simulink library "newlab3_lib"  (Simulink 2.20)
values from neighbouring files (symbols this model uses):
  h = 0.05    [initlab3.m]
undefined symbols (not defined in the file or in its folder): A, AIno, AOno, B, C, D, R, S, T, Ts, Xo

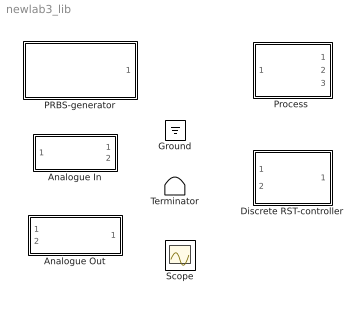
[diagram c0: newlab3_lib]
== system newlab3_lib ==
  Analogue In : Subsystem  mask(AnalogueIOBlock){h=h, AIno=AIno}
      mask prompts: h "Sample period"; AIno "Input port number"
      mask help: Analogue input block for use on PC running Linux.
  Analogue Out : Subsystem  mask(AnalogueIOBlock){h=h, AOno=AOno}
      mask prompts: h "Sample period"; AOno "Output port number"
      mask help: Analogue output block for use on PC running Linux
  Discrete RST-controller : Subsystem  mask(ControllerMaskBlock){R=R, S=S, T=T, h=h}
      mask prompts: R "R-polynomial"; S "S-polynomial"; T "T-polynomial"; h "Sample period"
      mask help: Discrete RST-controller (forward shift) R(q)u = -S(q)y + T(q)y_ref
  Ground : Ground
  PRBS-generator : Subsystem  mask(PRBSblockMask){h=h, N=5, Amp=2, offset=0, seed=0}
      mask prompts: h "Sample time (h)"; N "PRBS period (N)"; Amp "Amplitude"; seed "Random seed"
      mask help: A (P)RBS-generator
  "Process " : Subsystem  mask(SIMO Process){AOu=0, AIy=0, AIu=1, h=h}
      mask prompts: AOu "AO  u"; AIy "AI y"; AIu "AI u"; h "Sample Period"
      mask help: Process communication block. For use with Linux on PC with I/O.
  Scope : Scope
  Terminator : Terminator

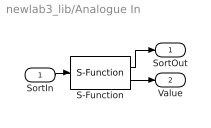
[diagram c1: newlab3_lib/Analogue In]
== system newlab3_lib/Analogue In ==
  SortIn : Inport  Port=1  PortWidth=-1  SampleTime=-1
  S-Function : S-Function  FunctionName=analogin  Parameters=h AIno  PortCounts=[]  SFunctionModules=''
  SortOut : Outport  Port=1  InitialOutput=0
  Value : Outport  Port=2  InitialOutput=0
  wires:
  S-Function/2 -> Value/1
  SortIn/1 -> S-Function/1
  S-Function/1 -> SortOut/1

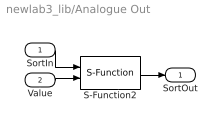
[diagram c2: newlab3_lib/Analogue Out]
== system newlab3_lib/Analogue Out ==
  SortIn : Inport  Port=1  PortWidth=-1  SampleTime=-1
  Value : Inport  Port=2  PortWidth=-1  SampleTime=-1
  S-Function2 : S-Function  FunctionName=analogout  Parameters=h AOno  PortCounts=[]  SFunctionModules=''
  SortOut : Outport  Port=1  InitialOutput=0
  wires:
  Value/1 -> S-Function2/2
  S-Function2/1 -> SortOut/1
  SortIn/1 -> S-Function2/1

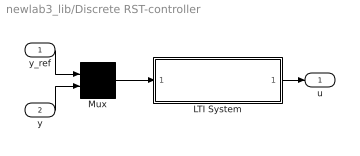
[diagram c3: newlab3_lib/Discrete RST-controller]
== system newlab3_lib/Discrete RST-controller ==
  y_ref : Inport  Port=1  PortWidth=-1  SampleTime=-1
  y : Inport  Port=2  PortWidth=-1  SampleTime=-1
  LTI System : Subsystem  mask(LTI Block){sys=ss(tf({T, -S},{R,R},h)), IC=0}
      mask prompts: sys "LTI system variable"; IC "Initial states   (state space only)"
      mask help: The LTI System Block accepts both continuous and discrete LTI objects as defined in the Control System Toolbox. Transfer function, state space, and zero/pole/gain formats are all supported in this block. Note: For multi-input systems, the input delays must be either all positive or all zero. Note: Initial states are only meaningful for state-space systems.
      mask init:
      | sysname='xxx';
      | [A,B,C,D,Xo,Td,Ts,sysname]=ltimask( 'InitializeVars',gcb,sys,IC,&1,&2);
      | ltimask( 'UpdateDiagram',gcb,sys,Td);
  Mux : Mux  Inputs=2
  u : Outport  Port=1  InitialOutput=0
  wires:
  y/1 -> Mux/2
  LTI System/1(Out1) -> u/1
  y_ref/1 -> Mux/1
  Mux/1 -> LTI System/1(In1)

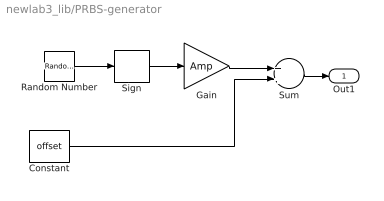
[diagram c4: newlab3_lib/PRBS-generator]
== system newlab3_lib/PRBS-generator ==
  Constant : Constant  Value=offset
  Gain : Gain  Gain=Amp
  Random Number : RandomNumber  Mean=0  Variance=1  Seed=seed  SampleTime=h*N
  Sign : Signum
  Sum : Sum  Inputs=++
  Out1 : Outport  Port=1  InitialOutput=0
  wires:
  Random Number/1 -> Sign/1
  Sign/1 -> Gain/1
  Gain/1 -> Sum/1
  Constant/1 -> Sum/2
  Sum/1 -> Out1/1

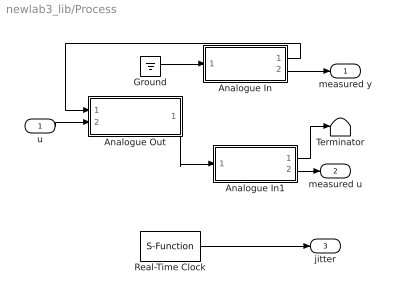
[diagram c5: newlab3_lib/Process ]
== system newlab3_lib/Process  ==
  u : Inport  Port=1  PortWidth=-1  SampleTime=-1
  Analogue In : Subsystem  mask(AnalogueIOBlock){h=h, AIy=AIy}
      mask prompts: h "Sample period"; AIy "Input port number"
      mask help: Analogue input block for use on PC running Linux.
  Analogue In1 : Subsystem  mask(AnalogueIOBlock){h=h, AIu=AIu}
      mask prompts: h "Sample period"; AIu "Input port number"
      mask help: Analogue input block for use on PC running Linux.
  Analogue Out : Subsystem  mask(AnalogueIOBlock){h=h, AOu=AOu}
      mask prompts: h "Sample period"; AOu "Output port number"
      mask help: Analogue output block for use on PC running Linux
  Ground : Ground
  Real-Time Clock : S-Function  FunctionName=timer  Parameters=h  PortCounts=[]  SFunctionModules=''
  Terminator : Terminator
  measured y : Outport  Port=1
  measured u : Outport  Port=2
  jitter : Outport  Port=3
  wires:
  Analogue In/1(SortOut) -> Analogue Out/1(SortIn)
  u/1 -> Analogue Out/2(Value)
  Real-Time Clock/1 -> jitter/1
  Analogue In/2(Value) -> measured y/1
  Ground/1 -> Analogue In/1(SortIn)
  Analogue In1/1(SortOut) -> Terminator/1
  Analogue In1/2(Value) -> measured u/1
  Analogue Out/1(SortOut) -> Analogue In1/1(SortIn)

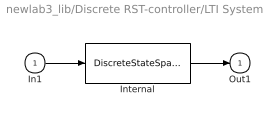
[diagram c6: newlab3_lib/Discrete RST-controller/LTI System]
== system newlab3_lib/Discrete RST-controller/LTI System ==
  In1 : Inport  Port=1  PortWidth=-1  SampleTime=-1
  Internal : DiscreteStateSpace  A=A  B=B  C=C  D=D  X0=Xo  SampleTime=Ts
  Out1 : Outport  Port=1  InitialOutput=0
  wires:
  In1/1 -> Internal/1
  Internal/1 -> Out1/1

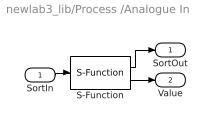
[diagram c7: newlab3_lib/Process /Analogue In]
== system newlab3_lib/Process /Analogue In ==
  SortIn : Inport  Port=1  PortWidth=-1  SampleTime=-1
  S-Function : S-Function  FunctionName=analogin  Parameters=h AIy  PortCounts=[]  SFunctionModules=''
  SortOut : Outport  Port=1  InitialOutput=0
  Value : Outport  Port=2  InitialOutput=0
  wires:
  S-Function/1 -> SortOut/1
  SortIn/1 -> S-Function/1
  S-Function/2 -> Value/1

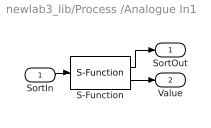
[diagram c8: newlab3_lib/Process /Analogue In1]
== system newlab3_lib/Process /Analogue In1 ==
  SortIn : Inport  Port=1  PortWidth=-1  SampleTime=-1
  S-Function : S-Function  FunctionName=analogin  Parameters=h AIu  PortCounts=[]  SFunctionModules=''
  SortOut : Outport  Port=1  InitialOutput=0
  Value : Outport  Port=2  InitialOutput=0
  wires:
  S-Function/2 -> Value/1
  SortIn/1 -> S-Function/1
  S-Function/1 -> SortOut/1

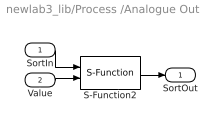
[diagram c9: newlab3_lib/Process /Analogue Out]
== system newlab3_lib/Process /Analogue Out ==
  SortIn : Inport  Port=1  PortWidth=-1  SampleTime=-1
  Value : Inport  Port=2  PortWidth=-1  SampleTime=-1
  S-Function2 : S-Function  FunctionName=analogout  Parameters=h AOu  PortCounts=[]  SFunctionModules=''
  SortOut : Outport  Port=1  InitialOutput=0
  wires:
  SortIn/1 -> S-Function2/1
  S-Function2/1 -> SortOut/1
  Value/1 -> S-Function2/2
